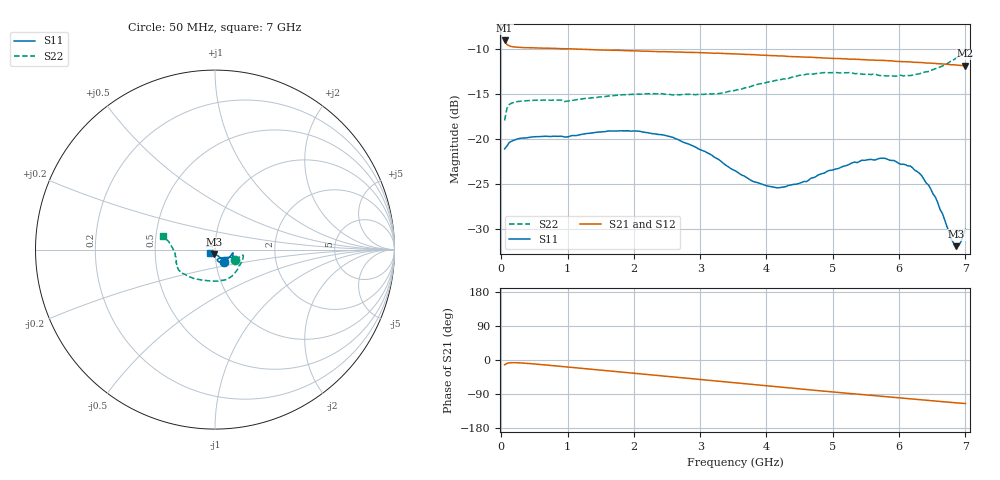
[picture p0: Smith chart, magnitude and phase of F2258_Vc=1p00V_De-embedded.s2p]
! Integrated Device Technology
! Corporate Headquarters
! 6024 Silver Creek Valley Road
! San Jose, CA 95138  USA
! Phone:  1-408-284-8200
! Toll Free:  1-800-223-1366
! Webpage:  http://www.idt.com/
! Timing and RF Division
! 515 Groton Road, Suite 102
! Westford, MA 01886-6024
! Device:  F2258
! Description: Voltage Variable RF Attenuator
! Frequency:  50.0 -  6000.00 MHz
! Package:  3x3 mm Thin QFN Plastic Package: 16 pin
! Ports:  2 RF, 2 DC
!  Pin  1  = NC
!  Pin  2  = NC
!  Pin  3  = RF2  = Port 2
!  Pin  4  = GND
!  Pin  5  = Vdd
!  Pin  6  = NC
!  Pin  7  = VCTRL
!  Pin  8  = NC
!  Pin  9  = GND
!  Pin 10  = RF1  = Port 1
!  Pin 11  = NC
!  Pin 12  = NC
!  Pin 13  = NC
!  Pin 14  = NC
!  Pin 15  = NC
!  Pin 16  = NC
! Vcntrl:  1.000 Volts
! Vdd:  +3.300 Volts
! Current:  1.156 mA
! Data:  The device was measured on a the F2258 evaluation board which has
!  individual transmission lines to the RF pins.  Data was collected
!  using a calibrated network analyzer.  The evaluation board was
!  de-embedded using a TRL calibration technique.
!  The reference plane is the edge of the package pin.
! Misc:  SN 10
!  Action Tracker AT0285
! Date Measured:  2014-12-10
! Date:  2016-01-13  MJV
! Note:
!  Integrated Device Technology supplies this data as a sample of measured
!  data at the package pin for this product.  Your particular data for this
!  product may vary.
!  Data was taken at 25 degrees C.
!  Integrated Device Technology reserves the right to change this data at anytime.
!Freq_(GHz)  S11M_(dB)  S11P_(deg)  S21M_(dB)  S21P_(deg)  S12M_(dB)  S12P_(deg)  S22M_(dB)  S22P_(deg)
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# GHz S dB R 50
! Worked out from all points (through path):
!   201 points, 50 MHz to 7 GHz, reference 50 ohm
!   highest |S21| = -9.11 dB at 50 MHz (marker M1); lowest = -11.9 dB at 7 GHz (marker M2)
!   group delay of S21, straight-line fit = 44.9 ps
!   lowest |S11| = -31.9 dB at 6.861 GHz (marker M3), VSWR 1.05, Z = 49.2 - j2.41 ohm
!   |S11| at or under -10 dB: start of sweep to end of sweep
!   |S22| runs from -18.0 to -10.4 dB; largest |S21 - S12| = 0.0014
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0.05  -21.12 -53.8  -9.11 -12.6  -9.11 -12.6  -17.97 -26.7
0.08475  -20.81 -27.9  -9.56 -8.9  -9.55 -8.9  -16.63 -14.6
0.189  -20.17 -12.8  -9.83 -7.0  -9.82 -7.0  -15.97 -11.2
1.2315  -19.48 -19.3  -10.08 -22.3  -10.09 -22.3  -15.56 -41.2
1.89175  -19.12 -22.3  -10.23 -33.1  -10.25 -33.1  -15.13 -58.8
2.37825  -19.53 -23.9  -10.35 -41.0  -10.34 -41.0  -15.01 -72.2
2.58675  -19.84 -25.6  -10.37 -44.5  -10.38 -44.5  -15.15 -78.4
3.07325  -21.41 -30.6  -10.47 -52.6  -10.50 -52.6  -15.06 -96.0
3.525  -23.53 -41.5  -10.60 -60.3  -10.61 -60.3  -14.64 -114.2
3.803  -24.75 -53.5  -10.68 -65.0  -10.71 -64.9  -14.10 -124.8
4.1505  -25.42 -66.5  -10.80 -70.7  -10.82 -70.6  -13.52 -135.2
4.60225  -24.75 -77.4  -10.96 -78.0  -10.98 -78.0  -12.84 -145.7
4.7065  -24.31 -76.9  -10.99 -79.7  -11.02 -79.6  -12.83 -147.7
5.43625  -22.38 -68.2  -11.23 -91.1  -11.25 -91.0  -12.84 -159.1
5.85325  -22.37 -59.9  -11.36 -97.6  -11.38 -97.5  -13.02 -167.5
6.166  -23.01 -56.6  -11.48 -102.4  -11.51 -102.3  -13.01 -174.8
6.33975  -24.07 -55.3  -11.56 -105.2  -11.58 -105.1  -12.73 -179.7
6.54825  -26.47 -59.3  -11.65 -108.3  -11.69 -108.3  -12.24 175.1
6.7915  -31.18 -88.2  -11.80 -111.9  -11.81 -111.8  -11.34 169.1
6.861  -31.90 -106.2  -11.83 -113.0  -11.85 -112.9  -11.07 167.8
6.9305  -31.44 -126.9  -11.87 -113.9  -11.90 -113.8  -10.77 166.8
7  -30.04 -147.7  -11.90 -114.9  -11.92 -114.9  -10.39 165.1
